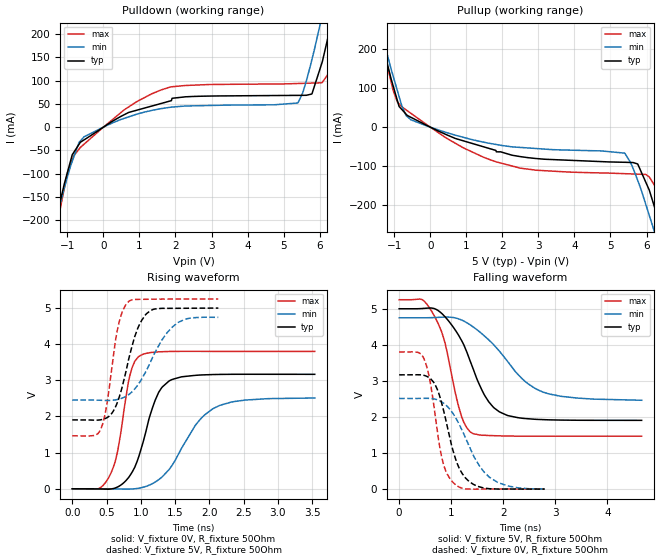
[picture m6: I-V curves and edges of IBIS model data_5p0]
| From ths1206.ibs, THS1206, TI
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|   data_5p0 Model
[Model]   data_5p0
Model_type   Output
Polarity   Non-Inverting
Vmeas = 2.5
Vref = 2.5
Cref = 2pF
Rref = 50
|   typ   min   max
|   (nom PVT)   (fast PVT)   (slow PVT)
C_comp   1.842e-12   1.842e-12   1.903e-12
|ON state : BUFFER OUTPUT TURNED HIGH
|C_comp   1.842e-12   1.842e-12   1.903e-12
|OFF state: BUFFER OUTPUT TURNED LOW
|C_comp   1.650e-12   1.642e-12   1.693e-12
| Where nom  PVT is Nominal Process, 5V, 43C
|   Fast PVT is Strong Process,  5.25V, -55C
|   Slow PVT is Weak Process,   4.75V, 145C
[Voltage Range]   5   4.75   5.25
|Ambient Temperature   25   125   -55
|Junction Temperature
[Temperature Range]   43   145   -55
[Pullup Reference]   5   4.75   5.25
[Pulldown Reference]   0   0   0
[Power Clamp Reference]   5   4.75   5.25
[GND Clamp Reference]   0   0   0
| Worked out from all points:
|   slope of the pulldown table from 0 to 0.75 V, typ, clamps not added: 23 ohm
|   slope of the pullup table from 0 to 0.75 V, typ, clamps not added: 24.5 ohm
|   falling waveform, V_fixture 5V, R_fixture 50Ohm: 20-80 % time 583ps typ, 874ps min, 378ps max; typ from 5 V to 1.91 V
|   rising waveform, V_fixture 0V, R_fixture 50Ohm: 20-80 % time 309ps typ, 515ps min, 202ps max; typ from 0 V to 3.17 V
|   rising waveform, V_fixture 5V, R_fixture 50Ohm: 20-80 % time 261ps typ, 401ps min, 176ps max; typ from 1.91 V to 5 V
|   falling waveform, V_fixture 0V, R_fixture 50Ohm: 20-80 % time 350ps typ, 543ps min, 252ps max; typ from 3.17 V to 0 V
[Pulldown]
|   Voltage   I(typ)   I(min)   I(max)
-5V       -1.6A      -1.47A     -1.792A
-1.306V   -194.6mA   -195.9mA   -216.2mA
-997.5mV  -96.96mA   -106.4mA   -98.24mA
-674.5mV  -36.59mA   -32.65mA   -46.93mA
924mV     36.29mA    27.74mA    54.61mA
1.906V    61.88mA    43.05mA    86.62mA
5.391V    68.1mA     51.72mA    93.56mA
5.785V    71.13mA    145mA      94.47mA
6.053V    135.5mA    233.8mA    95.09mA
6.3V      215.7mA    317mA      131.6mA
6.557V    306.2mA    403.9mA    221.8mA
10V       1.65A      1.705A     1.602A
[Pullup]
|   Voltage   I(typ)   I(min)   I(max)
-5V       1.695A     1.642A     1.754A
-2.617V   721.6mA    716.1mA    752.1mA
-1.31V    206.2mA    227.6mA    202.5mA
-913.5mV  68.42mA    93.77mA    64.66mA
-674.5mV  33.6mA     30.11mA    44.55mA
251.7mV   -11.2mA    -7.988mA   -15.95mA
2.499V    -75.61mA   -52.06mA   -105.3mA
5.391V    -90.16mA   -66.64mA   -119.4mA
5.755V    -94.57mA   -136.8mA   -120.6mA
6.216V    -203.5mA   -267.3mA   -148.4mA
6.557V    -312.2mA   -366.7mA   -263.9mA
10V       -1.605A    -1.56A     -1.695A
[Ramp]
R_load = 50
|   typ   min   max
dV/dt_r   1.90041/3.06568e-10   1.5075/5.13337e-10   2.28117/2.01302e-10
dV/dt_f   1.85651/5.8109e-10   1.37681/8.7855e-10   2.27022/3.76094e-10
[Falling Waveform]
V_fixture = 5V
V_fixture_min = 4.75V
V_fixture_max = 5.25V
R_fixture = 50Ohm
|   Time   V(typ)   V(min)   V(max)
0s        5V         4.75V      5.25V
434ps     5.006V     4.749V     5.259V
666ps     5.008V     4.756V     4.826V
878ps     4.782V     4.768V     4.067V
1.194ns   4.132V     4.691V     2.032V
1.434ns   3.284V     4.483V     1.528V
1.724ns   2.414V     4.132V     1.484V
2.082ns   2.039V     3.54V      1.471V
2.872ns   1.92V      2.64V      1.466V
4.656ns   1.906V     2.463V     1.466V
[Rising Waveform]
V_fixture = 0V
V_fixture_min = 0V
V_fixture_max = 0V
R_fixture = 50Ohm
|   Time   V(typ)   V(min)   V(max)
0s        1.91nV     4.517nV    1.571nV
536ps     -10.72mV   -1.868mV   324.7mV
658ps     45.93mV    -5.42mV    1.007V
842ps     364.7mV    -8.641mV   3.145V
982ps     956.7mV    18.93mV    3.675V
1.21ns    2.448V     184.8mV    3.781V
1.428ns   2.998V     569mV      3.8V
1.798ns   3.139V     1.759V     3.803V
2.15ns    3.164V     2.305V     3.802V
3.54ns    3.167V     2.512V     3.802V
[Rising Waveform]
V_fixture = 5V
V_fixture_min = 4.75V
V_fixture_max = 5.25V
R_fixture = 50Ohm
|   Time   V(typ)   V(min)   V(max)
0s        1.906V     2.455V     1.466V
418ps     1.909V     2.449V     1.655V
506ps     1.966V     2.444V     2.349V
656ps     2.379V     2.469V     4.37V
806ps     3.435V     2.584V     5.152V
958ps     4.449V     2.874V     5.241V
1.144ns   4.931V     3.514V     5.245V
1.316ns   4.993V     4.138V     5.249V
1.546ns   4.994V     4.601V     5.25V
2.132ns   5V         4.744V     5.25V
[Falling Waveform]
V_fixture = 0V
V_fixture_min = 0V
V_fixture_max = 0V
R_fixture = 50Ohm
|   Time   V(typ)   V(min)   V(max)
0s        3.167V     2.513V     3.802V
478ps     3.153V     2.516V     3.608V
600ps     3.062V     2.513V     2.938V
816ps     2.386V     2.417V     887.5mV
920ps     1.761V     2.299V     422.4mV
1.054ns   969.2mV    2.051V     157.2mV
1.324ns   236.2mV    1.258V     3.351mV
1.724ns   10.9mV     340.2mV    469.2uV
2.088ns   1.455mV    86.22mV    276.2uV
2.794ns   336.1uV    1.432mV    155.5uV
